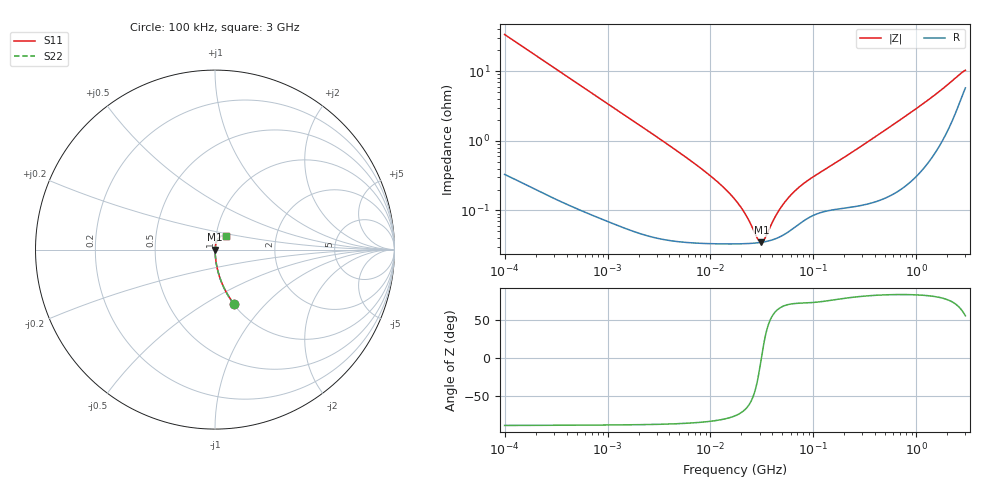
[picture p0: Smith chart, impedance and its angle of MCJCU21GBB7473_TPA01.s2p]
! MCJCU21GBB7473_TPA01  S-PARAMETER MODEL  ( Standard Model )
! Model Generated by TAIYO YUDEN Corporation (http://www.ty-top.com)
! Version 1.0
! TAIYO YUDEN Control No. 220601
! Copyright(c) 2015 TAIYO YUDEN CO.,LTD. All Rights Reserved.
! Product Description (link to TY-COMPAS)
! https://ds.yuden.co.jp/TYCOMPAS/or/detail?pn=MCJCU21GBB7473KTPA01&u=M
! Products Name : Multilayer Ceramic Capacitors
! Characteristics :
!  Capacitance : 0.047 [uF] , Rated Voltage : 50 [V] , TCC : X7R
!  Case Size : 2.0 x 1.25 / 0.079 x 0.049 [mm/inch] , Thickness : 1.25 / 0.049 [mm/inch]
!  (Conditions: Temperature = 25 [degC] , DC Bias Voltage = 0 [V])
! External Node Assignments :
!  1  o---| |---o  2
! GND o---------o GND
! Frequency Range : 100kHz  -  3GHz  [ 401 STEP ]
# MHZ S RI R 50
! Freq[MHz].  S11 Real  S11 Imag  S21 Real  S21 Imag  S12 Real  S12 Imag  S22 Real  S22 Imag
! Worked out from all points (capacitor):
!   401 points, 100 kHz to 3 GHz, reference 50 ohm
!   read as one part in series: C = 47 nF near 105.3 kHz
!   lowest |Z| = 34.9 mohm at 31.33 MHz (marker M1)
!   series resonance near 31.26 MHz, so ESL is about 550 pH
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0.1  0.1051 -0.3018  0.8949 0.3018  0.8949 0.3018  0.1051 -0.3018
0.147195  0.0526 -0.2178  0.9474 0.2178  0.9474 0.2178  0.0526 -0.2178
0.228123  0.0234 -0.1454  0.9766 0.1454  0.9766 0.1454  0.0234 -0.1454
0.562235  0.00467 -0.0605  0.9953 0.0605  0.9953 0.0605  0.00467 -0.0605
3.161081  0.000512 -0.0109  0.9995 0.0109  0.9995 0.0109  0.000512 -0.0109
6.178009  0.000374 -0.0054  0.9996 0.0054  0.9996 0.0054  0.000374 -0.0054
9.824692  0.000344 -0.00319  0.9997 0.00319  0.9997 0.00319  0.000344 -0.00319
13.7349  0.000335 -0.00205  0.9997 0.00205  0.9997 0.00205  0.000335 -0.00205
17.7727  0.000333 -0.00133  0.9997 0.00133  0.9997 0.00133  0.000333 -0.00133
22.41241  0.000335 -0.00076  0.9997 0.00076  0.9997 0.00076  0.000335 -0.00076
29.00125  0.000343 -0.000169  0.9997 0.000169  0.9997 0.000169  0.000343 -0.000169
31.3325  0.000349 5.52e-06  0.9997 -5.52e-06  0.9997 -5.52e-06  0.000349 5.52e-06
33.85116  0.000355 0.000181  0.9996 -0.000181  0.9996 -0.000181  0.000355 0.000181
42.68829  0.000392 0.000718  0.9996 -0.000718  0.9996 -0.000718  0.000392 0.000718
47.32384  0.000419 0.000967  0.9996 -0.000967  0.9996 -0.000967  0.000419 0.000967
53.83243  0.000466 0.00129  0.9995 -0.00129  0.9995 -0.00129  0.000466 0.00129
69.65816  0.000612 0.00195  0.9994 -0.00195  0.9994 -0.00195  0.000612 0.00195
97.38194  0.000842 0.00286  0.9992 -0.00286  0.9992 -0.00286  0.000842 0.00286
547.5153  0.00184 0.0156  0.9982 -0.0156  0.9982 -0.0156  0.00184 0.0156
1791.7  0.0128 0.0535  0.9872 -0.0535  0.9872 -0.0535  0.0128 0.0535
2637.286  0.0404 0.0771  0.9596 -0.0771  0.9596 -0.0771  0.0404 0.0771
3000  0.0608 0.0765  0.9392 -0.0765  0.9392 -0.0765  0.0608 0.0765
